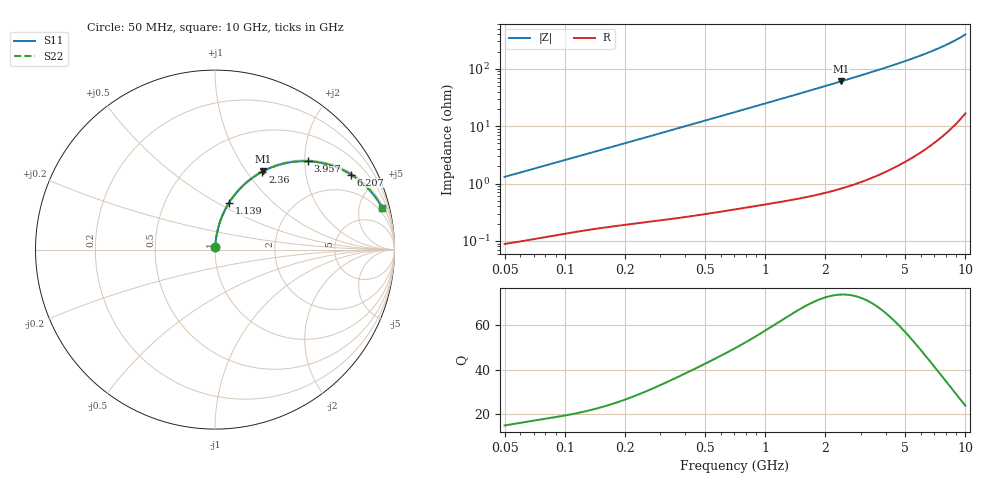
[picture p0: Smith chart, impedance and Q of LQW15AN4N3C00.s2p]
!Murata Part Number: LQW15AN4N3C00
!These Parameters are Measured in Series Mode Connection
!  o--[Z]--o
!Port1  Port2
!  o-------o
!Freq. Start=50[MHz] Stop=10[GHz], 401[Steps]
# Hz S RI R 50
!Freq.(Hz)	S 11(Real)	S 11(Imag)	S 21(Real)	S 21(Imag)	S 12(Real)	S 12(Imag)	S 22(Real)	S 22(Imag)
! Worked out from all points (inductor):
!   401 points, 50 MHz to 10 GHz, reference 50 ohm
!   read as one part in series: L = 4.13 nH near 51.34 MHz
!   highest Q = 74 at 2.392 GHz (marker M1), where L = 4.01 nH
!   S11 on the Smith chart (normalised r, x): 50 MHz: 1.00, +0.03; 1.139 GHz: 1.01, +0.57; 2.36 GHz: 1.02, +1.19; 3.957 GHz: 1.03, +2.07; 6.207 GHz: 1.08, +3.58; 10 GHz: 1.33, +7.92
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5e7  0.00106 0.013  0.9989 -0.013  0.9989 -0.013  0.00106 0.013
1.214486e8  0.00245 0.0309  0.9976 -0.0309  0.9976 -0.0309  0.00245 0.0309
1.956524e8  0.00431 0.0491  0.9957 -0.0491  0.9957 -0.0491  0.00431 0.0491
2.949953e8  0.00767 0.0733  0.9923 -0.0733  0.9923 -0.0733  0.00767 0.0733
4.689809e8  0.0162 0.1149  0.9838 -0.1149  0.9838 -0.1149  0.0162 0.1149
7.071068e8  0.0333 0.1695  0.9667 -0.1695  0.9667 -0.1695  0.0333 0.1695
9.094607e8  0.0521 0.2135  0.9479 -0.2135  0.9479 -0.2135  0.0521 0.2135
1.139142e9  0.0779 0.26  0.9221 -0.26  0.9221 -0.26  0.0779 0.26
1.408053e9  0.1131 0.3093  0.8869 -0.3093  0.8869 -0.3093  0.1131 0.3093
1.717543e9  0.1589 0.3585  0.8411 -0.3585  0.8411 -0.3585  0.1589 0.3585
2.013439e9  0.2062 0.3978  0.7938 -0.3978  0.7938 -0.3978  0.2062 0.3978
2.360312e9  0.2641 0.4341  0.7359 -0.4341  0.7359 -0.4341  0.2641 0.4341
2.391784e9  0.2694 0.4369  0.7306 -0.4369  0.7306 -0.4369  0.2694 0.4369
3.117263e9  0.3904 0.4809  0.6096 -0.4809  0.6096 -0.4809  0.3904 0.4809
3.956578e9  0.5177 0.4922  0.4823 -0.4922  0.4823 -0.4922  0.5177 0.4922
4.171863e9  0.5471 0.4901  0.4529 -0.4901  0.4529 -0.4901  0.5471 0.4901
5.088839e9  0.6564 0.4661  0.3436 -0.4661  0.3436 -0.4661  0.6564 0.4661
6.207365e9  0.7576 0.4181  0.2424 -0.4181  0.2424 -0.4181  0.7576 0.4181
7.086521e9  0.817 0.3746  0.183 -0.3746  0.183 -0.3746  0.817 0.3746
7.983737e9  0.8635 0.3293  0.1365 -0.3293  0.1365 -0.3293  0.8635 0.3293
8.759398e9  0.8947 0.2908  0.1053 -0.2908  0.1053 -0.2908  0.8947 0.2908
1e10  0.9315 0.2323  0.0685 -0.2323  0.0685 -0.2323  0.9315 0.2323
